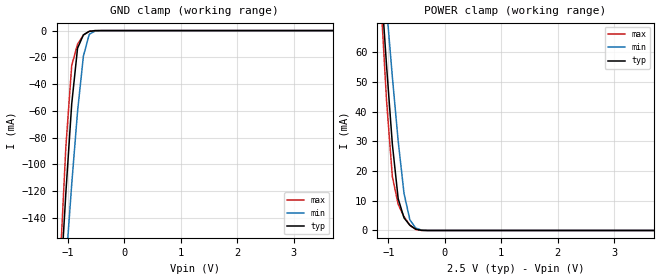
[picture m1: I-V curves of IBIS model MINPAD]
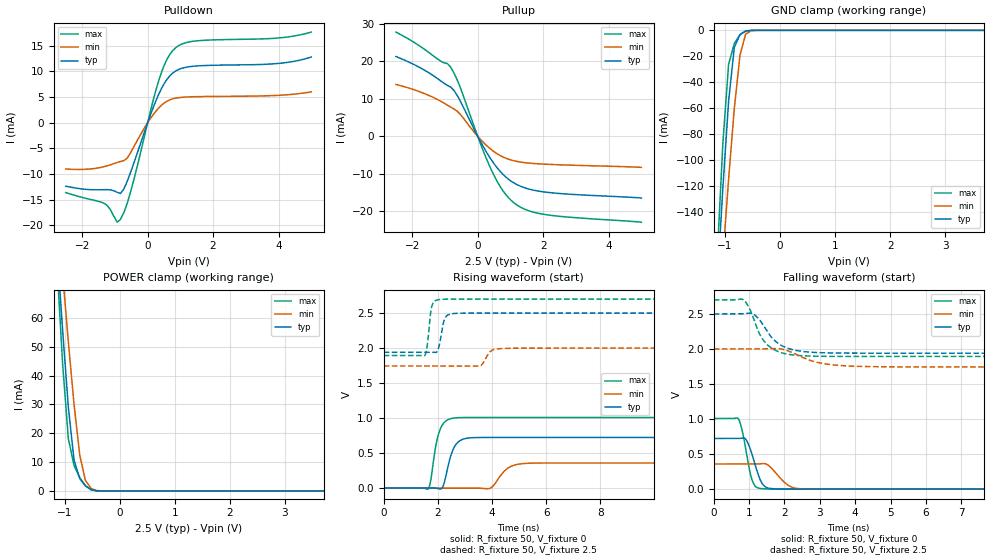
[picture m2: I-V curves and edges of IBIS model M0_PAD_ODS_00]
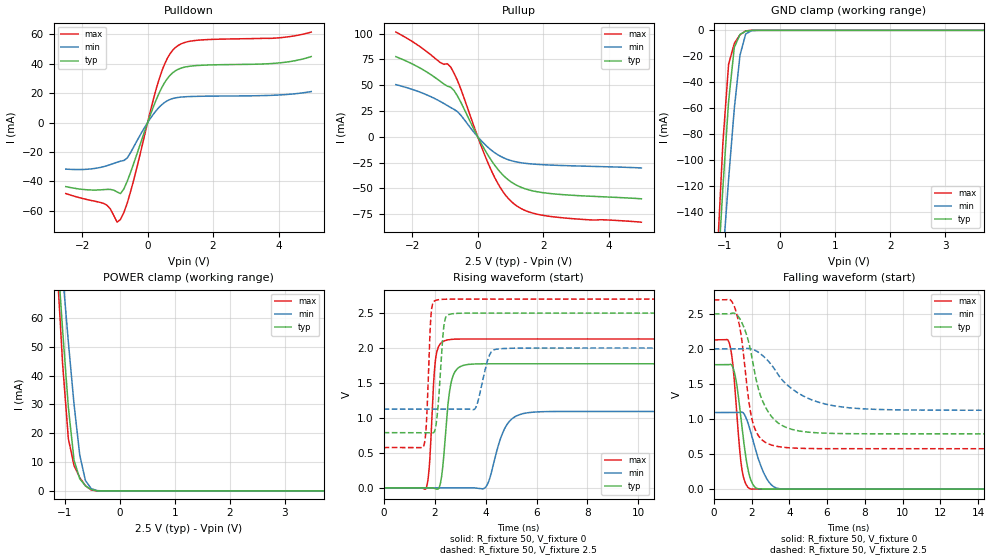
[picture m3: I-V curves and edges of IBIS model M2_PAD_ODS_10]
|   Microsemi Corporation
|   SmartFusion2 Automotive IBIS Model
[IBIS ver]   5.0
[File name]   as30208cg_25v_rev1p0.ibs
[File Rev]   1.0
[Date]   Wed Jul 17 2024
[Source] Simulated Models ONLY.
   All data is based on Spice simulation. All performed at Microsemi Corporation.
   Please refer to the Microsemi website for future updates at www.microsemi.com
[Notes]  Microsemi SmartFusion2 IBIS models for automotive operating conditions
   for DDRIO IO Banks IO Configurations ONLY. Models uses a software default
   fixed codes except for DDR3/SSTL15 which will always require calibrated
   codes.
   Automotive Temperature Grade 2 (t2) models cover a temperature range from
   -40C to 125C.
   Please refer to msio_auto_t2.ibs for MSIO IO Banks IO Configurations.
   Please refer to msiod_auto_t2.ibs for MSIOD IO Banks IO Configurations.
   The package parasitics of various package types are given.
   Uncomment the appropriate package or refer to the .pkg for specific
   per pin parasitic data.
   There are warnings related to non-monotonic and Increasing/Decreasing Current.
   They are expected on 20 Ohms and 30 Ohms I/O ODT models in DDR3/SSTL15.
[Disclaimer] This information is for board design considerations.
   Simulation based V/I curves contained in this model file are
   considered preliminary until verified against bench
   measurements. Maximum currents may vary from part to part but
   should not exceed maximum I/V curves provided in this model file.
[Copyright]  (c) 2015, Microsemi Corporation, All Rights Reserved.
| IBIS MODEL CHECKLIST
| Microsemi is dedicated to releasing quality IBIS models to customers.
| The following items have been
| verified for this IBIS model before release:
| 1)  Checked IBIS model by the golden parser ibischk5 [Complete]
| 2)  Ensured no errors reported by golden parser
|   for the IBIS model [Complete]
| 3)  Defined Vinl and Vinh for recievers [Complete]
| 4)  Defined Standard Load and Vmeas values for drivers [Complete]
| 5)  Defined overshoots for drivers and recievers [NA]
| 6)  Validated Ramp Values[Complete]
| 7)  Defined V-T Tables for all output drivers [Complete]
| 8)  Validated [Diff Pins] []
| 9)  Verified Package Parasitics [Complete]
| 10) Defined Standard Load Parameters and Specifications
|   for waveforms [Complete]
| 11) Defined and Validate Pin mappings [Complete]
| 12) Verified Ccomp Value []
| 13) Visually Inspected I-V Curves and V-T Tables  [Complete]
| 14) Presented Typ/Min/Max Values in the correct order for
|   all tables and parameters [Complete]
| 15) Simulated all output models with standard load and
|   switching through Vmeas [Complete]
| 16) Simulated all reciever models  [Complete]
| 17) Validated Models selectors. []
| 18) Visually inspected Spice and IBIS correlation for
|   a) Typical VT Curves [Complete]
|   b) Minimum VT Curves [Complete]
|   c) Maximum VT Curves [Complete]
| 19) Visually inspected Silicon and IBIS correlation
|   a) Typical IV Pull UP/ Pull Down Curves []
|   b) Minimum IV Pull UP/ Pull Down Curves []
|   c) Maximum IV Pull UP/ Pull Down Curves []
|   Component SmartFusion2
[Component]   SmartFusion2 W MRAM
[Manufacturer]   Avalanche Technology
[Package]
|  Design die-package: BGA
| variable   typ   min   max
R_pkg   0.72029   0.51528   1.0002
L_pkg   5.797e-9   4.155e-9   8.073e-9
C_pkg   1.116e-12   7.907e-13   1.753e-12
|Pin and Model info
[Pin]  signal_name  model_name   R_pin   L_pin   C_pin
L9   CS1#   MINPAD   0.4340		15.2000E-9		1.2600E-12
J10   CS2#   MINPAD   0.3800		13.5000E-9		1.0400E-12
K9   CLK1   MINPAD   0.4300		12.7000E-9		0.9790E-12
K8   CLK2   MINPAD   0.4480		14.6000E-9		1.1600E-12
M10   IO_0   MIOPAD   0.4010		12.4000E-9		1.2500E-12
M9   IO_1   MIOPAD   0.4050		14.2000E-9		1.1100E-12
L11   IO_2   MIOPAD   0.3780		11.8000E-9		1.2000E-12
M11   IO_3   MIOPAD   0.3700		11.8000E-9		1.2600E-12
M12   IO_4   MIOPAD   0.3710		11.1000E-9		1.1000E-12
N10   IO_5   MIOPAD   0.4050		13.8000E-9		1.1600E-12
N9   IO_6   MIOPAD   0.3830		15.2000E-9		1.0900E-12
N8   IO_7   MIOPAD   0.4480		16.4000E-9		1.0800E-12
J14   HTBSEL   MINPAD   0.1380		6.1700E-9		0.6060E-12
H14   HBP_2   MINPAD   0.1470		6.3900E-9		1.0000E-12
G13   HBP_1   MINPAD   0.1910		8.5000E-9		1.1500E-12
G12   HBP_0   MINPAD   0.2050		8.6800E-9		1.4200E-12
J11   RESET#   MINPAD   0.3410		14.1000E-9		1.6300E-12
J12   INT1#   MIOPAD   0.3080		12.5000E-9		1.2100E-12
K10   INT2#   MIOPAD   0.2120		10.3000E-9		0.8230E-12
M7   VSSIO   GND   NA   NA   NA
H8   VSSIO   GND   NA   NA   NA
L8   VSSIO   GND   NA   NA   NA
P10   VSSIO   GND   NA   NA   NA
H12   VSSIO   GND   NA   NA   NA
N12   VSSIO   GND   NA   NA   NA
P12   VSSIO   GND   NA   NA   NA
H13   VSSIO   GND   NA   NA   NA
N13   VSSIO   GND   NA   NA   NA
A3   VSS   GND   NA   NA   NA
B3   VSS   GND   NA   NA   NA
W3   VSS   GND   NA   NA   NA
Y3   VSS   GND   NA   NA   NA
A4   VSS   GND   NA   NA   NA
Y4   VSS   GND   NA   NA   NA
F5   VSS   GND   NA   NA   NA
G5   VSS   GND   NA   NA   NA
P5   VSS   GND   NA   NA   NA
R5   VSS   GND   NA   NA   NA
F6   VSS   GND   NA   NA   NA
H6   VSS   GND   NA   NA   NA
J6   VSS   GND   NA   NA   NA
L6   VSS   GND   NA   NA   NA
N6   VSS   GND   NA   NA   NA
R6   VSS   GND   NA   NA   NA
L7   VSS   GND   NA   NA   NA
N7   VSS   GND   NA   NA   NA
G8   VSS   GND   NA   NA   NA
P8   VSS   GND   NA   NA   NA
G10   VSS   GND   NA   NA   NA
H10   VSS   GND   NA   NA   NA
L12   VSS   GND   NA   NA   NA
L13   VSS   GND   NA   NA   NA
P13   VSS   GND   NA   NA   NA
F14   VSS   GND   NA   NA   NA
L14   VSS   GND   NA   NA   NA
N14   VSS   GND   NA   NA   NA
R14   VSS   GND   NA   NA   NA
F15   VSS   GND   NA   NA   NA
G15   VSS   GND   NA   NA   NA
P15   VSS   GND   NA   NA   NA
R15   VSS   GND   NA   NA   NA
A16   VSS   GND   NA   NA   NA
Y16   VSS   GND   NA   NA   NA
A17   VSS   GND   NA   NA   NA
B17   VSS   GND   NA   NA   NA
W17   VSS   GND   NA   NA   NA
Y17   VSS   GND   NA   NA   NA
G6   VCCIO   POWER   NA   NA   NA
P6   VCCIO   POWER   NA   NA   NA
G7   VCCIO   POWER   NA   NA   NA
J7   VCCIO   POWER   NA   NA   NA
P7   VCCIO   POWER   NA   NA   NA
M8   VCCIO   POWER   NA   NA   NA
H9   VCCIO   POWER   NA   NA   NA
H11   VCCIO   POWER   NA   NA   NA
N11   VCCIO   POWER   NA   NA   NA
J13   VCCIO   POWER   NA   NA   NA
M13   VCCIO   POWER   NA   NA   NA
G14   VCCIO   POWER   NA   NA   NA
P14   VCCIO   POWER   NA   NA   NA
K6   VCC   POWER   NA   NA   NA
M6   VCC   POWER   NA   NA   NA
K7   VCC   POWER   NA   NA   NA
G9   VCC   POWER   NA   NA   NA
P9   VCC   POWER   NA   NA   NA
G11   VCC   POWER   NA   NA   NA
K11   VCC   POWER   NA   NA   NA
P11   VCC   POWER   NA   NA   NA
K13   VCC   POWER   NA   NA   NA
K14   VCC   POWER   NA   NA   NA
M14   VCC   POWER   NA   NA   NA
K12   VDD   POWER   NA   NA   NA
| END PIN INFO
| IOPAD
[Model Selector] MIOPAD
| Model Description
M0_PAD_ODS_00   ODS_00
M1_PAD_ODS_01   ODS_01
M2_PAD_ODS_10   ODS_10
M3_PAD_ODS_11   ODS_11
| Models and submodels in the file (5): MINPAD (Input), M0_PAD_ODS_00 (I/O), M2_PAD_ODS_10 (I/O), M1_PAD_ODS_01 (I/O), M3_PAD_ODS_11 (I/O)
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| INPAD
[Model] MINPAD
Model_type Input
Enable   Active-High
Vinl  =  0.7
Vinh  =  1.8
| Capacitance   typ   min   max
C_comp   1.560802e-12  1.468911e-12  1.706460e-12
| Variables   typ   min   max
[GND Clamp Reference]   0   0   0
[POWER Clamp Reference]   2.5   2   2.7
[Pulldown Reference]   0   0   0
[Pullup Reference]   2.5   2   2.7
[Temperature Range]   25   125   -40
[Voltage Range]   2.5   2   2.7
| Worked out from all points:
|   GND clamp passes 1 mA (typ) near -0.64 V on its own axis
|   POWER clamp passes 1 mA (typ) near -0.56 V on its own axis
[GND Clamp]
| Voltage   I(typ)   I(min)   I(max)
-2.5V     -1.297A    -1.146A    -1.538A
-1.138V   -196mA     -238.3mA   -175.4mA
-1.034V   -121.2mA   -175.1mA   -86.75mA
-931mV    -54.83mA   -114.9mA   -26.2mA
-827.6mV  -13.18mA   -60.42mA   -10.12mA
-724.1mV  -3.225mA   -19.15mA   -3.367mA
-620.7mV  -622.7uA   -2.801mA   -432.6uA
-517.2mV  -35.11uA   -320.3uA   -7.266uA
-413.8mV  -840.2nA   -24.53uA   -57.27nA
5V        0A         0A         0A
[POWER Clamp]
| Voltage   I(typ)   I(min)   I(max)
-2.5V     511mA      454.9mA    606.6mA
-1.138V   84.76mA    99.9mA     78.64mA
-1.034V   55.67mA    75.27mA    43.94mA
-931mV    29.07mA    51.7mA     18.16mA
-827.6mV  10.68mA    30.08mA    8.788mA
-724.1mV  4.238mA    12.45mA    4.618mA
-620.7mV  1.771mA    3.587mA    1.776mA
-517.2mV  465uA      837.9uA    329.7uA
-413.8mV  47.65uA    120.2uA    11.19uA
-310.3mV  1.515uA    11.72uA    116.8nA
5V        0A         0A         0A
[Model] M0_PAD_ODS_00
Model_type I/O
Enable   Active-High
Vinl  =  0.7
Vinh  =  1.8
Vmeas =  1.25
Cref  =  30e-12
| Capacitance   typ   min   max
C_comp   1.569373e-12  1.477665e-12  1.713725e-12
| Variables   typ   min   max
[GND Clamp Reference]   0   0   0
[POWER Clamp Reference]   2.5   2   2.7
[Pulldown Reference]   0   0   0
[Pullup Reference]   2.5   2   2.7
[Temperature Range]   25   125   -40
[Voltage Range]   2.5   2   2.7
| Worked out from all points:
|   slope of the pulldown table from 0 to 0.375 V, typ, clamps not added: 62.2 ohm
|   slope of the pullup table from 0 to 0.375 V, typ, clamps not added: 65.8 ohm
|   GND clamp passes 1 mA (typ) near -0.64 V on its own axis
|   POWER clamp passes 1 mA (typ) near -0.56 V on its own axis
|   falling waveform, R_fixture 50, V_fixture 0: 20-80 % time 279ps typ, 407ps min, 228ps max; typ from 0.724 V to 0 V
|   falling waveform, R_fixture 50, V_fixture 2.5: 20-80 % time 573ps typ, 848ps min, 480ps max; typ from 2.5 V to 1.94 V
|   rising waveform, R_fixture 50, V_fixture 0: 20-80 % time 318ps typ, 469ps min, 281ps max; typ from 0 V to 0.724 V
|   rising waveform, R_fixture 50, V_fixture 2.5: 20-80 % time 166ps typ, 247ps min, 131ps max; typ from 1.94 V to 2.5 V
[GND Clamp]
| Voltage   I(typ)   I(min)   I(max)
-2.5V     -1.297A    -1.146A    -1.538A
-1.138V   -196mA     -238.3mA   -175.4mA
-1.034V   -121.2mA   -175.1mA   -86.76mA
-931mV    -54.83mA   -114.9mA   -26.21mA
-827.6mV  -13.18mA   -60.42mA   -10.12mA
-724.1mV  -3.226mA   -19.15mA   -3.372mA
-620.7mV  -623.1uA   -2.801mA   -433.9uA
-517.2mV  -35.15uA   -320.3uA   -7.309uA
-413.8mV  -841.1nA   -24.53uA   -57.63nA
5V        0A         0A         0A
[POWER Clamp]
| Voltage   I(typ)   I(min)   I(max)
-2.5V     511mA      454.9mA    606.6mA
-1.138V   84.76mA    99.9mA     78.64mA
-1.034V   55.67mA    75.27mA    43.94mA
-931mV    29.07mA    51.7mA     18.16mA
-827.6mV  10.68mA    30.08mA    8.788mA
-724.1mV  4.238mA    12.45mA    4.618mA
-620.7mV  1.771mA    3.587mA    1.776mA
-517.2mV  465uA      837.9uA    329.7uA
-413.8mV  47.65uA    120.2uA    11.19uA
-310.3mV  1.515uA    11.72uA    116.8nA
5V        0A         0A         0A
[Pulldown]
| Voltage   I(typ)   I(min)   I(max)
-2.5V     -12.35mA   -9.004mA   -13.6mA
-1.345V   -13.04mA   -8.57mA    -15.65mA
-1.138V   -13.07mA   -8.191mA   -16.91mA
-931mV    -13.55mA   -7.74mA    -19.37mA
-827.6mV  -13.78mA   -7.539mA   -18.82mA
-517.2mV  -9.616mA   -5.796mA   -13.4mA
344.8mV   5.633mA    2.926mA    8.322mA
603.4mV   8.558mA    4.247mA    12.51mA
948.3mV   10.39mA    4.896mA    15.04mA
1.638V    11.13mA    5.111mA    16.04mA
3.99V     11.57mA    5.352mA    16.53mA
5V        12.82mA    6.029mA    17.68mA
[Pullup]
| Voltage   I(typ)   I(min)   I(max)
-2.5V     21.3mA     13.86mA    27.83mA
-1.552V   17.28mA    11.15mA    22.76mA
-827.6mV  13.17mA    7.825mA    18.5mA
-724.1mV  12.26mA    7.304mA    16.87mA
-517.2mV  9.175mA    5.726mA    12.68mA
86.21mV   -1.417mA   -831.8uA   -2.006mA
431mV     -6.444mA   -3.64mA    -9.217mA
775.9mV   -10.17mA   -5.503mA   -14.57mA
1.121V    -12.49mA   -6.527mA   -17.82mA
1.552V    -14.02mA   -7.108mA   -19.81mA
2.069V    -14.86mA   -7.416mA   -20.85mA
5V        -16.43mA   -8.255mA   -22.89mA
[Ramp]
dV/dt_r   0.434162/0.318029n  0.215384/0.469462n  0.605568/0.280922n
dV/dt_f   0.335983/0.573041n  0.153621/0.848321n  0.483841/0.479587n
R_load = 50
[Falling Waveform]
R_fixture = 50
V_fixture = 0
V_fixture_min = 0
V_fixture_max = 0
| Time   V(typ)   V(min)   V(max)
0s        723.6mV    359mV      1.009V
700.2ps   724.5mV    359.4mV    999.5mV
799.5ps   727.6mV    359.5mV    844.4mV
898.7ps   715.8mV    359.6mV    590.4mV
1.081ns   498.3mV    359.7mV    134.8mV
1.193ns   311mV      359.7mV    33.04mV
1.376ns   76.94mV    363.9mV    6.935mV
2.11ns    1.08mV     52.76mV    499.8uV
2.526ns   303uV      4.236mV    80.06uV
21.88ns   -155.3nV   483.7nV    -32.69nV
[Falling Waveform]
R_fixture = 50
V_fixture = 2.5
V_fixture_min = 2
V_fixture_max = 2.7
| Time   V(typ)   V(min)   V(max)
0s        2.5V       2V         2.7V
838.4ps   2.502V     2V         2.703V
1.131ns   2.495V     2.001V     2.432V
1.287ns   2.419V     2.001V     2.222V
1.466ns   2.289V     2.003V     2.086V
1.843ns   2.072V     2.004V     1.959V
2.373ns   1.975V     1.913V     1.908V
3.12ns    1.945V     1.79V      1.895V
4.48ns    1.94V      1.748V     1.894V
21.88ns   1.94V      1.744V     1.894V
[Rising Waveform]
R_fixture = 50
V_fixture = 0
V_fixture_min = 0
V_fixture_max = 0
| Time   V(typ)   V(min)   V(max)
0s        3.691nV    84.17nV    -49.53nV
1.643ns   -227.3uV   -358.4uV   -11.64mV
1.944ns   -1.334mV   -424.2uV   642.3mV
2.088ns   -13.51mV   -455.6uV   843.7mV
2.23ns    68.07mV    -486.5uV   936mV
2.641ns   607.3mV    -576.2uV   1.003V
3.895ns   723.5mV    -6.514mV   1.009V
4.598ns   723.6mV    289.1mV    1.009V
5.331ns   723.6mV    354.9mV    1.009V
21.88ns   723.6mV    359mV      1.009V
[Rising Waveform]
R_fixture = 50
V_fixture = 2.5
V_fixture_min = 2
V_fixture_max = 2.7
| Time   V(typ)   V(min)   V(max)
0s        1.94V      1.744V     1.894V
1.526ns   1.941V     1.744V     1.898V
1.774ns   1.941V     1.744V     2.595V
2.09ns    2.115V     1.745V     2.695V
2.281ns   2.44V      1.745V     2.699V
2.734ns   2.497V     1.745V     2.699V
3.549ns   2.499V     1.743V     2.699V
3.986ns   2.499V     1.966V     2.699V
4.579ns   2.499V     1.996V     2.699V
21.88ns   2.5V       2V         2.7V
[Model] M2_PAD_ODS_10
Model_type I/O
Enable   Active-High
Vinl  =  0.7
Vinh  =  1.8
Vmeas =  1.25
Cref  =  30e-12
| Capacitance   typ   min   max
C_comp   1.569373e-12  1.477665e-12  1.713725e-12
| Variables   typ   min   max
[GND Clamp Reference]   0   0   0
[POWER Clamp Reference]   2.5   2   2.7
[Pulldown Reference]   0   0   0
[Pullup Reference]   2.5   2   2.7
[Temperature Range]   25   125   -40
[Voltage Range]   2.5   2   2.7
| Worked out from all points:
|   slope of the pulldown table from 0 to 0.375 V, typ, clamps not added: 17.8 ohm
|   slope of the pullup table from 0 to 0.375 V, typ, clamps not added: 18 ohm
|   GND clamp passes 1 mA (typ) near -0.64 V on its own axis
|   POWER clamp passes 1 mA (typ) near -0.56 V on its own axis
|   falling waveform, R_fixture 50, V_fixture 0: 20-80 % time 504ps typ, 779ps min, 385ps max; typ from 1.77 V to 0 V
|   falling waveform, R_fixture 50, V_fixture 2.5: 20-80 % time 1.03ns typ, 2.06ns min, 617ps max; typ from 2.5 V to 0.789 V
|   rising waveform, R_fixture 50, V_fixture 0: 20-80 % time 269ps typ, 559ps min, 184ps max; typ from 0 V to 1.77 V
|   rising waveform, R_fixture 50, V_fixture 2.5: 20-80 % time 194ps typ, 336ps min, 137ps max; typ from 0.789 V to 2.5 V
[GND Clamp]
| Voltage   I(typ)   I(min)   I(max)
-2.5V     -1.297A    -1.146A    -1.538A
-1.138V   -196mA     -238.3mA   -175.4mA
-1.034V   -121.2mA   -175.1mA   -86.76mA
-931mV    -54.83mA   -114.9mA   -26.21mA
-827.6mV  -13.18mA   -60.42mA   -10.12mA
-724.1mV  -3.226mA   -19.15mA   -3.372mA
-620.7mV  -623.1uA   -2.801mA   -433.9uA
-517.2mV  -35.15uA   -320.3uA   -7.309uA
-413.8mV  -841.1nA   -24.53uA   -57.63nA
5V        0A         0A         0A
[POWER Clamp]
| Voltage   I(typ)   I(min)   I(max)
-2.5V     511mA      454.9mA    606.6mA
-1.138V   84.76mA    99.9mA     78.64mA
-1.034V   55.67mA    75.27mA    43.94mA
-931mV    29.07mA    51.7mA     18.16mA
-827.6mV  10.68mA    30.08mA    8.788mA
-724.1mV  4.238mA    12.45mA    4.618mA
-620.7mV  1.771mA    3.587mA    1.776mA
-517.2mV  465uA      837.9uA    329.7uA
-413.8mV  47.65uA    120.2uA    11.19uA
-310.3mV  1.515uA    11.72uA    116.8nA
5V        0A         0A         0A
[Pulldown]
| Voltage   I(typ)   I(min)   I(max)
-2.5V     -43.5mA    -31.6mA    -48.22mA
-1.345V   -45.55mA   -29.94mA   -54.89mA
-1.138V   -45.4mA    -28.55mA   -58.67mA
-931mV    -47.14mA   -26.9mA    -67.65mA
-827.6mV  -48.21mA   -26.21mA   -65.71mA
-517.2mV  -33.61mA   -20.26mA   -46.69mA
344.8mV   19.68mA    10.22mA    29mA
603.4mV   29.91mA    14.84mA    43.66mA
948.3mV   36.32mA    17.11mA    52.56mA
1.638V    38.89mA    17.86mA    56.1mA
3.99V     40.44mA    18.69mA    57.52mA
5V        44.82mA    21.06mA    61.44mA
[Pullup]
| Voltage   I(typ)   I(min)   I(max)
-2.5V     77.6mA     50.54mA    101.4mA
-1.552V   62.66mA    40.54mA    82.36mA
-1.138V   53.57mA    34.14mA    71.79mA
-827.6mV  48.05mA    28.38mA    67.64mA
-517.2mV  33.55mA    20.94mA    46.33mA
86.21mV   -5.181mA   -3.04mA    -7.328mA
431mV     -23.56mA   -13.31mA   -33.69mA
775.9mV   -37.17mA   -20.11mA   -53.29mA
1.121V    -45.67mA   -23.86mA   -65.22mA
1.552V    -51.29mA   -25.98mA   -72.55mA
2.155V    -54.68mA   -27.23mA   -76.79mA
5V        -59.99mA   -30.11mA   -82.63mA
[Ramp]
dV/dt_r   1.06496/0.269332n  0.655668/0.559175n  1.27778/0.184221n
dV/dt_f   1.02665/1.03253n  0.524479/2.05902n  1.27424/0.6168n
R_load = 50
[Falling Waveform]
R_fixture = 50
V_fixture = 0
V_fixture_min = 0
V_fixture_max = 0
| Time   V(typ)   V(min)   V(max)
0s        1.775V     1.093V     2.13V
857.3ps   1.78V      1.093V     2.05V
1.009ns   1.738V     1.093V     1.781V
1.158ns   1.587V     1.093V     1.302V
1.467ns   944.2mV    1.099V     327.1mV
1.898ns   185.7mV    869mV      8.061mV
2.174ns   30.86mV    601.8mV    2.134mV
2.651ns   2.232mV    229.1mV    813.3uV
3.494ns   858.2uV    5.952mV    777.6uV
21.88ns   425nV      1.228uV    2.027nV
[Falling Waveform]
R_fixture = 50
V_fixture = 2.5
V_fixture_min = 2
V_fixture_max = 2.7
| Time   V(typ)   V(min)   V(max)
0s        2.5V       2V         2.7V
1.093ns   2.508V     2.001V     2.603V
1.463ns   2.391V     2.001V     2.174V
1.819ns   2.128V     2.008V     1.331V
2.047ns   1.84V      1.996V     970.4mV
2.456ns   1.348V     1.935V     730mV
3.042ns   1.043V     1.778V     630.4mV
4.443ns   834.3mV    1.374V     583.8mV
6.686ns   792.8mV    1.176V     577.1mV
21.88ns   788.9mV    1.126V     576.3mV
[Rising Waveform]
R_fixture = 50
V_fixture = 0
V_fixture_min = 0
V_fixture_max = 0
| Time   V(typ)   V(min)   V(max)
0s        2.218nV    46.46nV    -54.5nV
1.669ns   -287.1uV   -373.2uV   -5.497mV
2.043ns   -13.92mV   -456.8uV   1.855V
2.275ns   162.4mV    -508.6uV   2.079V
2.472ns   984.4mV    -552.7uV   2.113V
2.926ns   1.715V     -654.2uV   2.128V
4.015ns   1.774V     14.5mV     2.129V
4.792ns   1.774V     876.7mV    2.129V
5.654ns   1.774V     1.074V     2.129V
21.88ns   1.775V     1.093V     2.13V
[Rising Waveform]
R_fixture = 50
V_fixture = 2.5
V_fixture_min = 2
V_fixture_max = 2.7
| Time   V(typ)   V(min)   V(max)
0s        788.9mV    1.126V     576.3mV
1.579ns   788.5mV    1.126V     605.5mV
1.683ns   788.5mV    1.126V     949.8mV
1.858ns   788.4mV    1.126V     2.472V
2.074ns   947.8mV    1.126V     2.685V
2.359ns   2.3V       1.127V     2.697V
2.623ns   2.485V     1.127V     2.699V
3.591ns   2.499V     1.133V     2.699V
4.504ns   2.499V     1.987V     2.699V
21.88ns   2.5V       2V         2.7V
